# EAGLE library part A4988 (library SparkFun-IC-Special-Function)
DMOS Microstepping Driver with Translator(IC-11483)
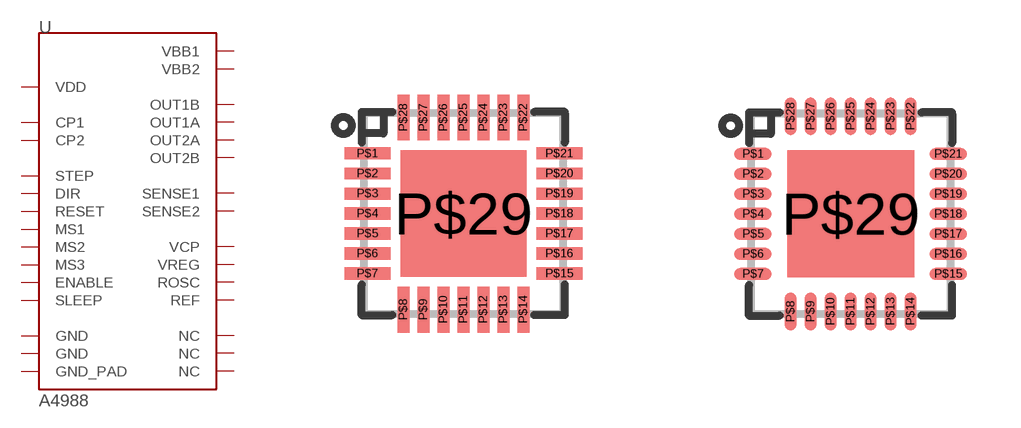
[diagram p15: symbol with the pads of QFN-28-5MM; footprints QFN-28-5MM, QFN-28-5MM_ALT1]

Designator prefix U

## A49885MM  [QFN-28-5MM]
P$1  OUT2B
P$2  ENABLE  in
P$3  GND  pwr
P$4  CP1
P$5  CP2
P$6  VCP
P$7  NC  nc
P$8  VREG
P$9  MS1  in
P$10  MS2  in
P$11  MS3  in
P$12  RESET  in
P$13  ROSC
P$14  SLEEP  in
P$15  VDD  pwr
P$16  STEP  in
P$17  REF
P$18  GND  pwr
P$19  DIR  in
P$20  NC  nc
P$21  OUT1B
P$22  VBB1
P$23  SENSE1
P$24  OUT1A
P$25  NC  nc
P$26  OUT2A
P$27  SENSE2
P$28  VBB2
P$29  GND_PAD  pwr

## A4988ALT1 (PROD_ID: IC-11483)  [QFN-28-5MM_ALT1]
Pads as for QFN-28-5MM

## A4988ALT2  [QFN-28-5MM_ALT2]
Pads as for QFN-28-5MM

## A49881:1  [QFN-28-5MM-1:1]
Pads as for QFN-28-5MM

## A4988ALT1_REDUCED_PASTE (PROD_ID: IC-11483)  [QFN-28-5MM_ALT1_REDUCED_PASTE]
Pads as for QFN-28-5MM

## Footprint QFN-28-5MM (pad centres in mm)
smd 1.15 x 0.3: P$1 -2.4,1.5; P$2 -2.4,1; P$3 -2.4,0.5; P$4 -2.4,0; P$5 -2.4,-0.5; P$6 -2.4,-1; P$7 -2.4,-1.5; P$15 2.4,-1.5; P$16 2.4,-1; P$17 2.4,-0.5; P$18 2.4,0; P$19 2.4,0.5; P$20 2.4,1; P$21 2.4,1.5
smd 0.3 x 1.15: P$8 -1.5,-2.4; P$9 -1,-2.4; P$10 -0.5,-2.4; P$11 0,-2.4; P$12 0.5,-2.4; P$13 1,-2.4; P$14 1.5,-2.4; P$22 1.5,2.4; P$23 1,2.4; P$24 0.5,2.4; P$25 0,2.4; P$26 -0.5,2.4; P$27 -1,2.4; P$28 -1.5,2.4
smd 3.15 x 3.15: P$29 0,0

## Footprint QFN-28-5MM_ALT1 (pad centres in mm)
smd 0.94 x 0.3: P$1 -2.44,1.5; P$2 -2.44,1; P$3 -2.44,0.5; P$4 -2.44,0; P$5 -2.44,-0.5; P$6 -2.44,-1; P$7 -2.44,-1.5; P$15 2.44,-1.5; P$16 2.44,-1; P$17 2.44,-0.5; P$18 2.44,0; P$19 2.44,0.5; P$20 2.44,1; P$21 2.44,1.5
smd 0.3 x 0.94: P$8 -1.5,-2.44; P$9 -1,-2.44; P$10 -0.5,-2.44; P$11 0,-2.44; P$12 0.5,-2.44; P$13 1,-2.44; P$14 1.5,-2.44; P$22 1.5,2.44; P$23 1,2.44; P$24 0.5,2.44; P$25 0,2.44; P$26 -0.5,2.44; P$27 -1,2.44; P$28 -1.5,2.44
smd 3.175 x 3.175: P$29 0,0

## Footprint QFN-28-5MM_ALT2 (pad centres in mm)
smd 0.889 x 0.28: P$1 -2.401,1.5; P$2 -2.401,1; P$3 -2.401,0.5; P$4 -2.401,0; P$5 -2.401,-0.5; P$6 -2.401,-1; P$7 -2.401,-1.5; P$15 2.401,-1.5; P$16 2.401,-1; P$17 2.401,-0.5; P$18 2.401,0; P$19 2.401,0.5; P$20 2.401,1; P$21 2.401,1.5
smd 0.28 x 0.889: P$8 -1.5,-2.401; P$9 -1,-2.401; P$10 -0.5,-2.401; P$11 0,-2.401; P$12 0.5,-2.401; P$13 1,-2.401; P$14 1.5,-2.401; P$22 1.5,2.401; P$23 1,2.401; P$24 0.5,2.401; P$25 0,2.401; P$26 -0.5,2.401; P$27 -1,2.401; P$28 -1.5,2.401
smd 3.048 x 3.048: P$29 0,0

## Footprint QFN-28-5MM-1:1 (pad centres in mm)
smd 1.15 x 0.3: P$1 -2.527,1.5; P$2 -2.527,1; P$3 -2.527,0.5; P$4 -2.527,0; P$5 -2.527,-0.5; P$6 -2.527,-1; P$7 -2.527,-1.5; P$15 2.527,-1.5; P$16 2.527,-1; P$17 2.527,-0.5; P$18 2.527,0; P$19 2.527,0.5; P$20 2.527,1; P$21 2.527,1.5
smd 0.3 x 1.15: P$8 -1.5,-2.527; P$9 -1,-2.527; P$10 -0.5,-2.527; P$11 0,-2.527; P$12 0.5,-2.527; P$13 1,-2.527; P$14 1.5,-2.527; P$22 1.5,2.527; P$23 1,2.527; P$24 0.5,2.527; P$25 0,2.527; P$26 -0.5,2.527; P$27 -1,2.527; P$28 -1.5,2.527
smd 3.15 x 3.15: P$29 0,0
